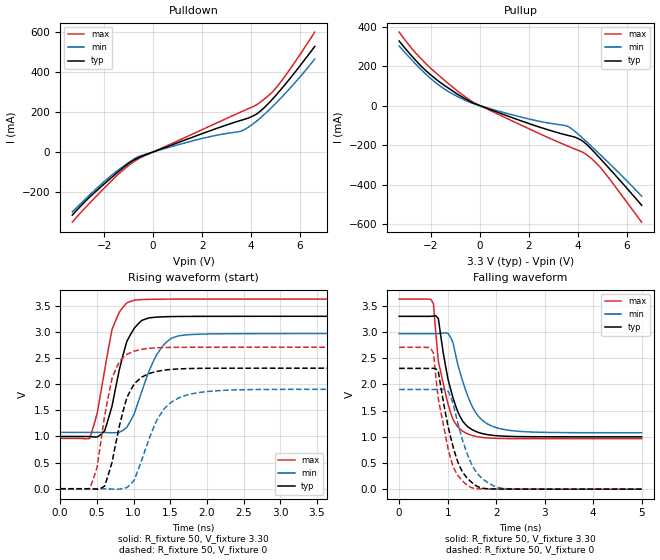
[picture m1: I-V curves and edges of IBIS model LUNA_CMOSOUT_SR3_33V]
[IBIS Ver]   3.2
[Comment Char]   |_char
[File name]   sg8201cja_33v_b.ibs
[File Rev]   1.1
[Date]   2021/10/19 9:35:58
[Source]
[Notes]
[Disclaimer]
This information is for modeling purposes only, and is not guaranteed.
Property of SEIKO EPSON Corp.,
unauthorized reproduction and/or distribution is strictly prohibited.
[Copyright]
Copyright 2021, SEIKO EPSON Corp.
[Component]   2G005_2016
Si_location Pin
Timing_location Pin
[Manufacturer]   SEIKO EPSON Corp.
| 2016 PKG
[Package]
R_pkg   25m   NA   NA
L_pkg   0.25n   NA   NA
C_pkg   0.183p   NA   NA
[Pin] signal_name   model_name
1   OE   NC
2   GND   GND
3   OUT   LUNA_CMOSOUT_SR3_33V
4   VCC   POWER
| Models and submodels in the file (1): LUNA_CMOSOUT_SR3_33V (Output)
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[Model]   LUNA_CMOSOUT_SR3_33V
Model_type Output
Polarity Non-Inverting
Vmeas=1.65
C_comp   2.5p   2.0p   3.0p
[Temperature Range] 25   140   -40
[Voltage Range]   3.30   2.97   3.63
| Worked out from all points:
|   slope of the pulldown table from 0 to 0.495 V, typ, clamps not added: 21.7 ohm
|   slope of the pullup table from 0 to 0.495 V, typ, clamps not added: 21.4 ohm
|   falling waveform, R_fixture 50, V_fixture 3.30: 20-80 % time 346ps typ, 426ps min, 304ps max; typ from 3.3 V to 1 V
|   falling waveform, R_fixture 50, V_fixture 0: 20-80 % time 357ps typ, 411ps min, 321ps max; typ from 2.31 V to 0 V
|   rising waveform, R_fixture 50, V_fixture 3.30: 20-80 % time 235ps typ, 314ps min, 210ps max; typ from 1 V to 3.3 V
|   rising waveform, R_fixture 50, V_fixture 0: 20-80 % time 248ps typ, 345ps min, 205ps max; typ from 0 V to 2.31 V
[Pullup]
-3.3V     327.1mA    301.9mA    372.3mA
-2.6V     225.8mA    207.4mA    263.2mA
-1.8V     134.3mA    115.4mA    165.7mA
-1.2V     81.28mA    65.11mA    102.6mA
-400mV    21.09mA    16.43mA    27.37mA
1.8V      -82.09mA   -61.55mA   -105.4mA
3.5V      -147.7mA   -101.4mA   -200.3mA
3.7V      -153.8mA   -113.3mA   -210.6mA
4V        -165.9mA   -143.2mA   -225.6mA
4.4V      -201.4mA   -188.3mA   -252.3mA
5V        -280.1mA   -258.8mA   -325.2mA
6.6V      -504.1mA   -458.2mA   -589.8mA
[Pulldown]
-3.3V     -315.7mA   -300mA     -351mA
-2.6V     -226.8mA   -215.9mA   -257.1mA
-1.8V     -138.6mA   -127.2mA   -156.5mA
-1.2V     -76.23mA   -70.27mA   -87.64mA
-700mV    -34.8mA    -29.41mA   -41.81mA
1.7V      77.96mA    58.11mA    94.58mA
3.6V      158.6mA    104.6mA    200.9mA
4.1V      181.3mA    142mA      227.9mA
4.5V      217.2mA    183.1mA    260.6mA
4.9V      267.6mA    229.8mA    303.6mA
5.2V      309.5mA    267.4mA    348.5mA
6.6V      527.6mA    464.7mA    599.3mA
[Falling Waveform]
R_fixture=50
V_fixture=3.30
V_fixture_min=2.97
V_fixture_max=3.63
0s        3.3V       2.97V      3.63V
656.6ps   3.302V     2.97V      3.624V
707.1ps   3.304V     2.969V     3.539V
808.1ps   3.259V     2.971V     2.444V
959.6ps   2.337V     2.985V     1.812V
1.111ns   1.743V     2.795V     1.328V
1.313ns   1.294V     2.051V     1.104V
1.616ns   1.089V     1.411V     1.001V
2.02ns    1.02V      1.171V     970.1mV
5ns       999.9mV    1.078V     963.5mV
[Falling Waveform]
R_fixture=50
V_fixture=0
V_fixture_min=0
V_fixture_max=0
0s        2.307V     1.903V     2.708V
606.1ps   2.306V     1.903V     2.704V
707.1ps   2.308V     1.902V     2.6V
808.1ps   2.239V     1.903V     1.72V
1.01ns    1.19V      1.87V      769.5mV
1.212ns   511.5mV    1.256V     259.3mV
1.414ns   200.7mV    648.1mV    67.28mV
1.667ns   31.56mV    244.9mV    5.958mV
2.071ns   2.717mV    27.5mV     1.233mV
5ns       263.4uV    460uV      161.2uV
[Rising Waveform]
R_fixture=50
V_fixture=3.30
V_fixture_min=2.97
V_fixture_max=3.63
0s        999.9mV    1.078V     963.5mV
404ps     998.8mV    1.078V     963.8mV
505.1ps   989.3mV    1.078V     1.443V
606.1ps   1.107V     1.077V     2.264V
707.1ps   1.58V      1.071V     3.045V
858.6ps   2.566V     1.121V     3.476V
959.6ps   2.951V     1.296V     3.585V
1.313ns   3.284V     2.559V     3.627V
1.616ns   3.297V     2.926V     3.629V
5ns       3.3V       2.97V      3.63V
[Rising Waveform]
R_fixture=50
V_fixture=0
V_fixture_min=0
V_fixture_max=0
0s        0V         0V         0V
404ps     -762.6uV   166.6uV    6.994mV
505.1ps   -8.282mV   353.5uV    416.7mV
606.1ps   50.56mV    -924.6uV   1.391V
757.6ps   860.6mV    -8.148mV   2.284V
909.1ps   1.743V     22.71mV    2.571V
1.01ns    2.007V     163mV      2.634V
1.364ns   2.257V     1.417V     2.7V
1.717ns   2.298V     1.789V     2.707V
5ns       2.307V     1.903V     2.708V
[Ramp]
R_load=50
dV/dt_r   1.384E+0/2.452E-10   1.142E+0/3.451E-10   1.625E+0/2.053E-10
dV/dt_f   1.380E+0/3.463E-10   1.135E+0/4.238E-10   1.600E+0/3.041E-10
|[End   LUNA_CMOSOUT_SR3_33V
